PROGRAM error_code
VAR
	alarm_type: WSTRING(INT#25);
	err: BOOL;
END_VAR
VAR // added by the converter: edge detectors and wires of the graphical bodies
    _w1 : BOOL;
END_VAR

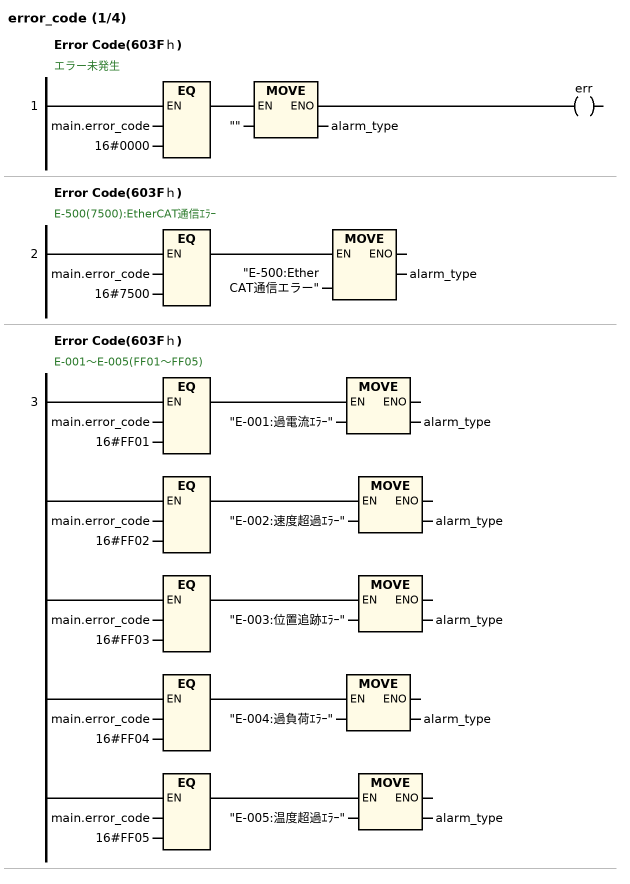
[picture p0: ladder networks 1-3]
// NETWORK 1: Error Code(603Fｈ)
// エラー未発生
_w1 := main.error_code = 16#0000;
IF _w1 THEN alarm_type := ""; END_IF
err := _w1;

// NETWORK 2: Error Code(603Fｈ)
// E-500(7500):EtherCAT通信ｴﾗｰ
IF main.error_code = 16#7500 THEN alarm_type := "E-500:EtherCAT通信エラー"; END_IF

// NETWORK 3: Error Code(603Fｈ)
// E-001～E-005(FF01～FF05)
IF main.error_code = 16#FF01 THEN alarm_type := "E-001:過電流ｴﾗｰ"; END_IF
IF main.error_code = 16#FF02 THEN alarm_type := "E-002:速度超過ｴﾗｰ"; END_IF
IF main.error_code = 16#FF03 THEN alarm_type := "E-003:位置追跡ｴﾗｰ"; END_IF
IF main.error_code = 16#FF04 THEN alarm_type := "E-004:過負荷ｴﾗｰ"; END_IF
IF main.error_code = 16#FF05 THEN alarm_type := "E-005:温度超過ｴﾗｰ"; END_IF

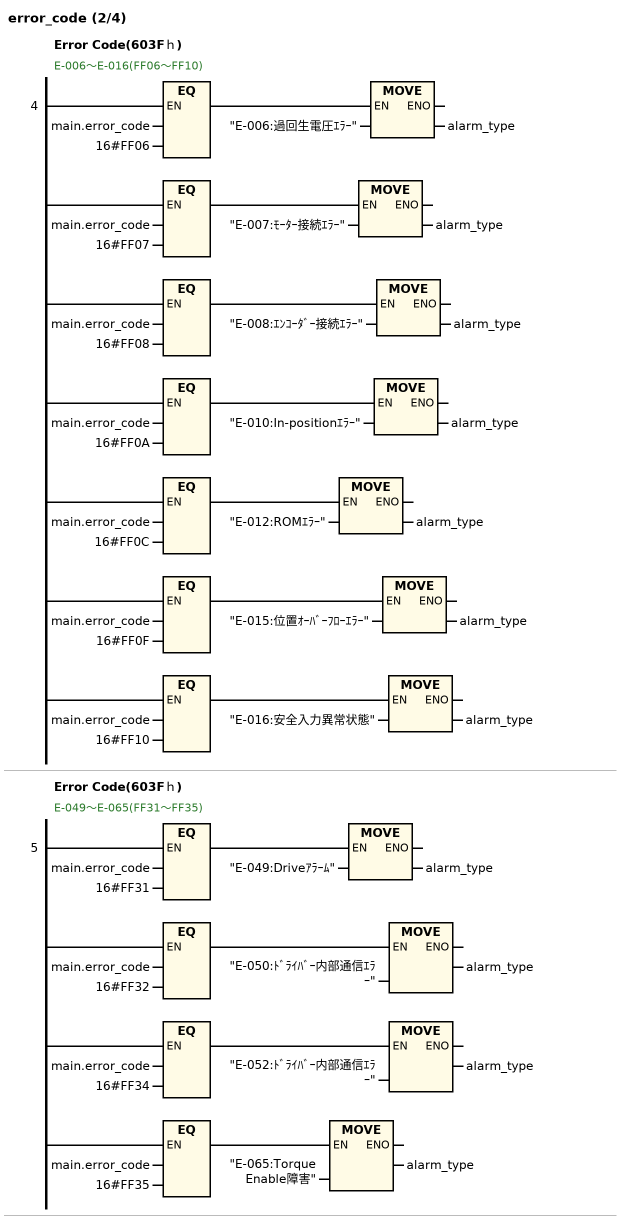
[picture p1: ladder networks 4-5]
// NETWORK 4: Error Code(603Fｈ)
// E-006～E-016(FF06～FF10)
IF main.error_code = 16#FF06 THEN alarm_type := "E-006:過回生電圧ｴﾗｰ"; END_IF
IF main.error_code = 16#FF07 THEN alarm_type := "E-007:ﾓｰﾀｰ接続ｴﾗｰ"; END_IF
IF main.error_code = 16#FF08 THEN alarm_type := "E-008:ｴﾝｺｰﾀﾞｰ接続ｴﾗｰ"; END_IF
IF main.error_code = 16#FF0A THEN alarm_type := "E-010:In-positionｴﾗｰ"; END_IF
IF main.error_code = 16#FF0C THEN alarm_type := "E-012:ROMｴﾗｰ"; END_IF
IF main.error_code = 16#FF0F THEN alarm_type := "E-015:位置ｵｰﾊﾞｰﾌﾛｰｴﾗｰ"; END_IF
IF main.error_code = 16#FF10 THEN alarm_type := "E-016:安全入力異常状態"; END_IF

// NETWORK 5: Error Code(603Fｈ)
// E-049～E-065(FF31～FF35)
IF main.error_code = 16#FF31 THEN alarm_type := "E-049:Driveｱﾗｰﾑ"; END_IF
IF main.error_code = 16#FF32 THEN alarm_type := "E-050:ﾄﾞﾗｲﾊﾞｰ内部通信ｴﾗｰ"; END_IF
IF main.error_code = 16#FF34 THEN alarm_type := "E-052:ﾄﾞﾗｲﾊﾞｰ内部通信ｴﾗｰ"; END_IF
IF main.error_code = 16#FF35 THEN alarm_type := "E-065:Torque Enable障害"; END_IF

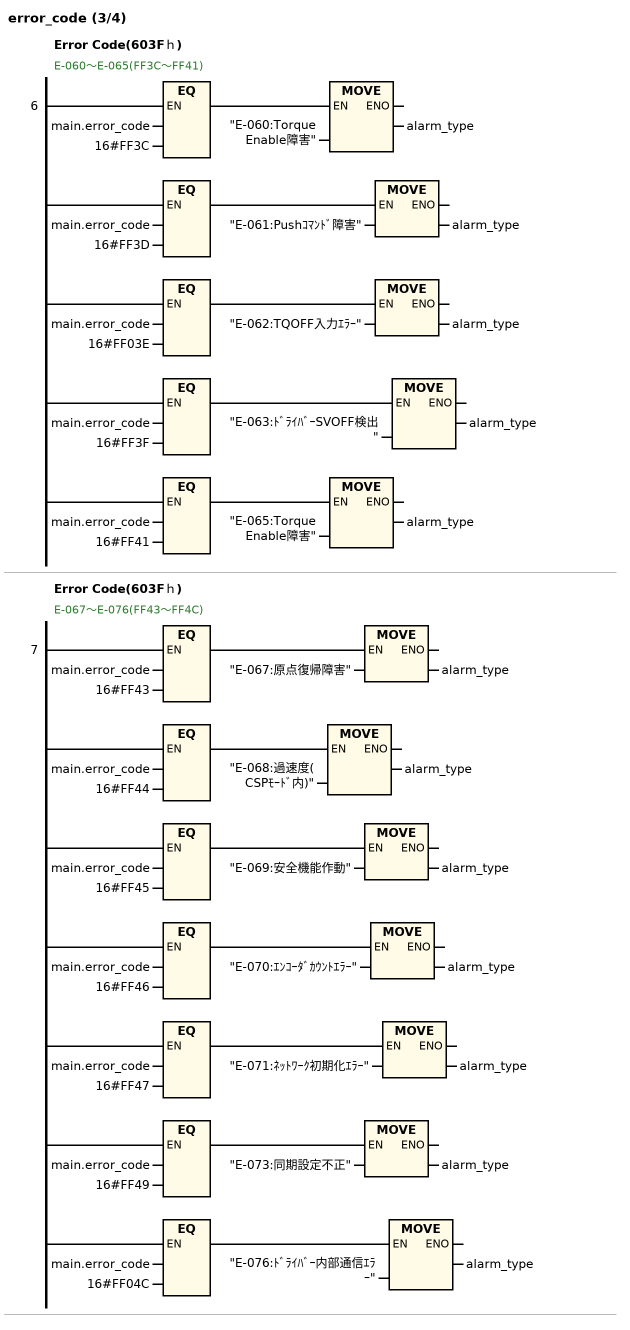
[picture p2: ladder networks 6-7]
// NETWORK 6: Error Code(603Fｈ)
// E-060～E-065(FF3C～FF41)
IF main.error_code = 16#FF3C THEN alarm_type := "E-060:Torque Enable障害"; END_IF
IF main.error_code = 16#FF3D THEN alarm_type := "E-061:Pushｺﾏﾝﾄﾞ障害"; END_IF
IF main.error_code = 16#FF03E THEN alarm_type := "E-062:TQOFF入力ｴﾗｰ"; END_IF
IF main.error_code = 16#FF3F THEN alarm_type := "E-063:ﾄﾞﾗｲﾊﾞｰSVOFF検出"; END_IF
IF main.error_code = 16#FF41 THEN alarm_type := "E-065:Torque Enable障害"; END_IF

// NETWORK 7: Error Code(603Fｈ)
// E-067～E-076(FF43～FF4C)
IF main.error_code = 16#FF43 THEN alarm_type := "E-067:原点復帰障害"; END_IF
IF main.error_code = 16#FF44 THEN alarm_type := "E-068:過速度(CSPﾓｰﾄﾞ内)"; END_IF
IF main.error_code = 16#FF45 THEN alarm_type := "E-069:安全機能作動"; END_IF
IF main.error_code = 16#FF46 THEN alarm_type := "E-070:ｴﾝｺｰﾀﾞｶｳﾝﾄｴﾗｰ"; END_IF
IF main.error_code = 16#FF47 THEN alarm_type := "E-071:ﾈｯﾄﾜｰｸ初期化ｴﾗｰ"; END_IF
IF main.error_code = 16#FF49 THEN alarm_type := "E-073:同期設定不正"; END_IF
IF main.error_code = 16#FF04C THEN alarm_type := "E-076:ﾄﾞﾗｲﾊﾞｰ内部通信ｴﾗｰ"; END_IF

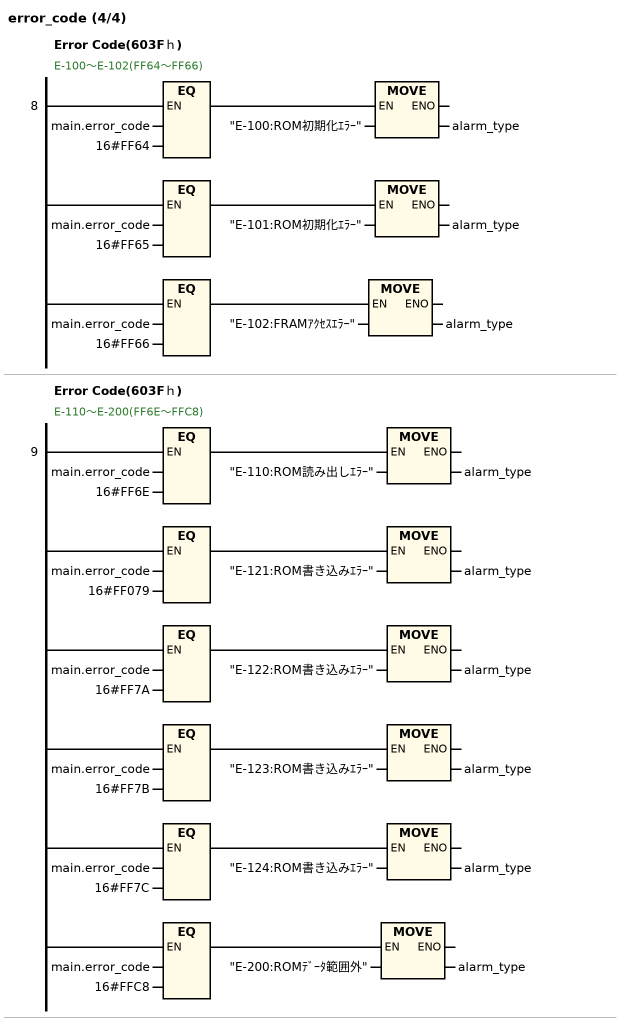
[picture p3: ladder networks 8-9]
// NETWORK 8: Error Code(603Fｈ)
// E-100～E-102(FF64～FF66)
IF main.error_code = 16#FF64 THEN alarm_type := "E-100:ROM初期化ｴﾗｰ"; END_IF
IF main.error_code = 16#FF65 THEN alarm_type := "E-101:ROM初期化ｴﾗｰ"; END_IF
IF main.error_code = 16#FF66 THEN alarm_type := "E-102:FRAMｱｸｾｽｴﾗｰ"; END_IF

// NETWORK 9: Error Code(603Fｈ)
// E-110～E-200(FF6E～FFC8)
IF main.error_code = 16#FF6E THEN alarm_type := "E-110:ROM読み出しｴﾗｰ"; END_IF
IF main.error_code = 16#FF079 THEN alarm_type := "E-121:ROM書き込みｴﾗｰ"; END_IF
IF main.error_code = 16#FF7A THEN alarm_type := "E-122:ROM書き込みｴﾗｰ"; END_IF
IF main.error_code = 16#FF7B THEN alarm_type := "E-123:ROM書き込みｴﾗｰ"; END_IF
IF main.error_code = 16#FF7C THEN alarm_type := "E-124:ROM書き込みｴﾗｰ"; END_IF
IF main.error_code = 16#FFC8 THEN alarm_type := "E-200:ROMﾃﾞｰﾀ範囲外"; END_IF

END_PROGRAM
